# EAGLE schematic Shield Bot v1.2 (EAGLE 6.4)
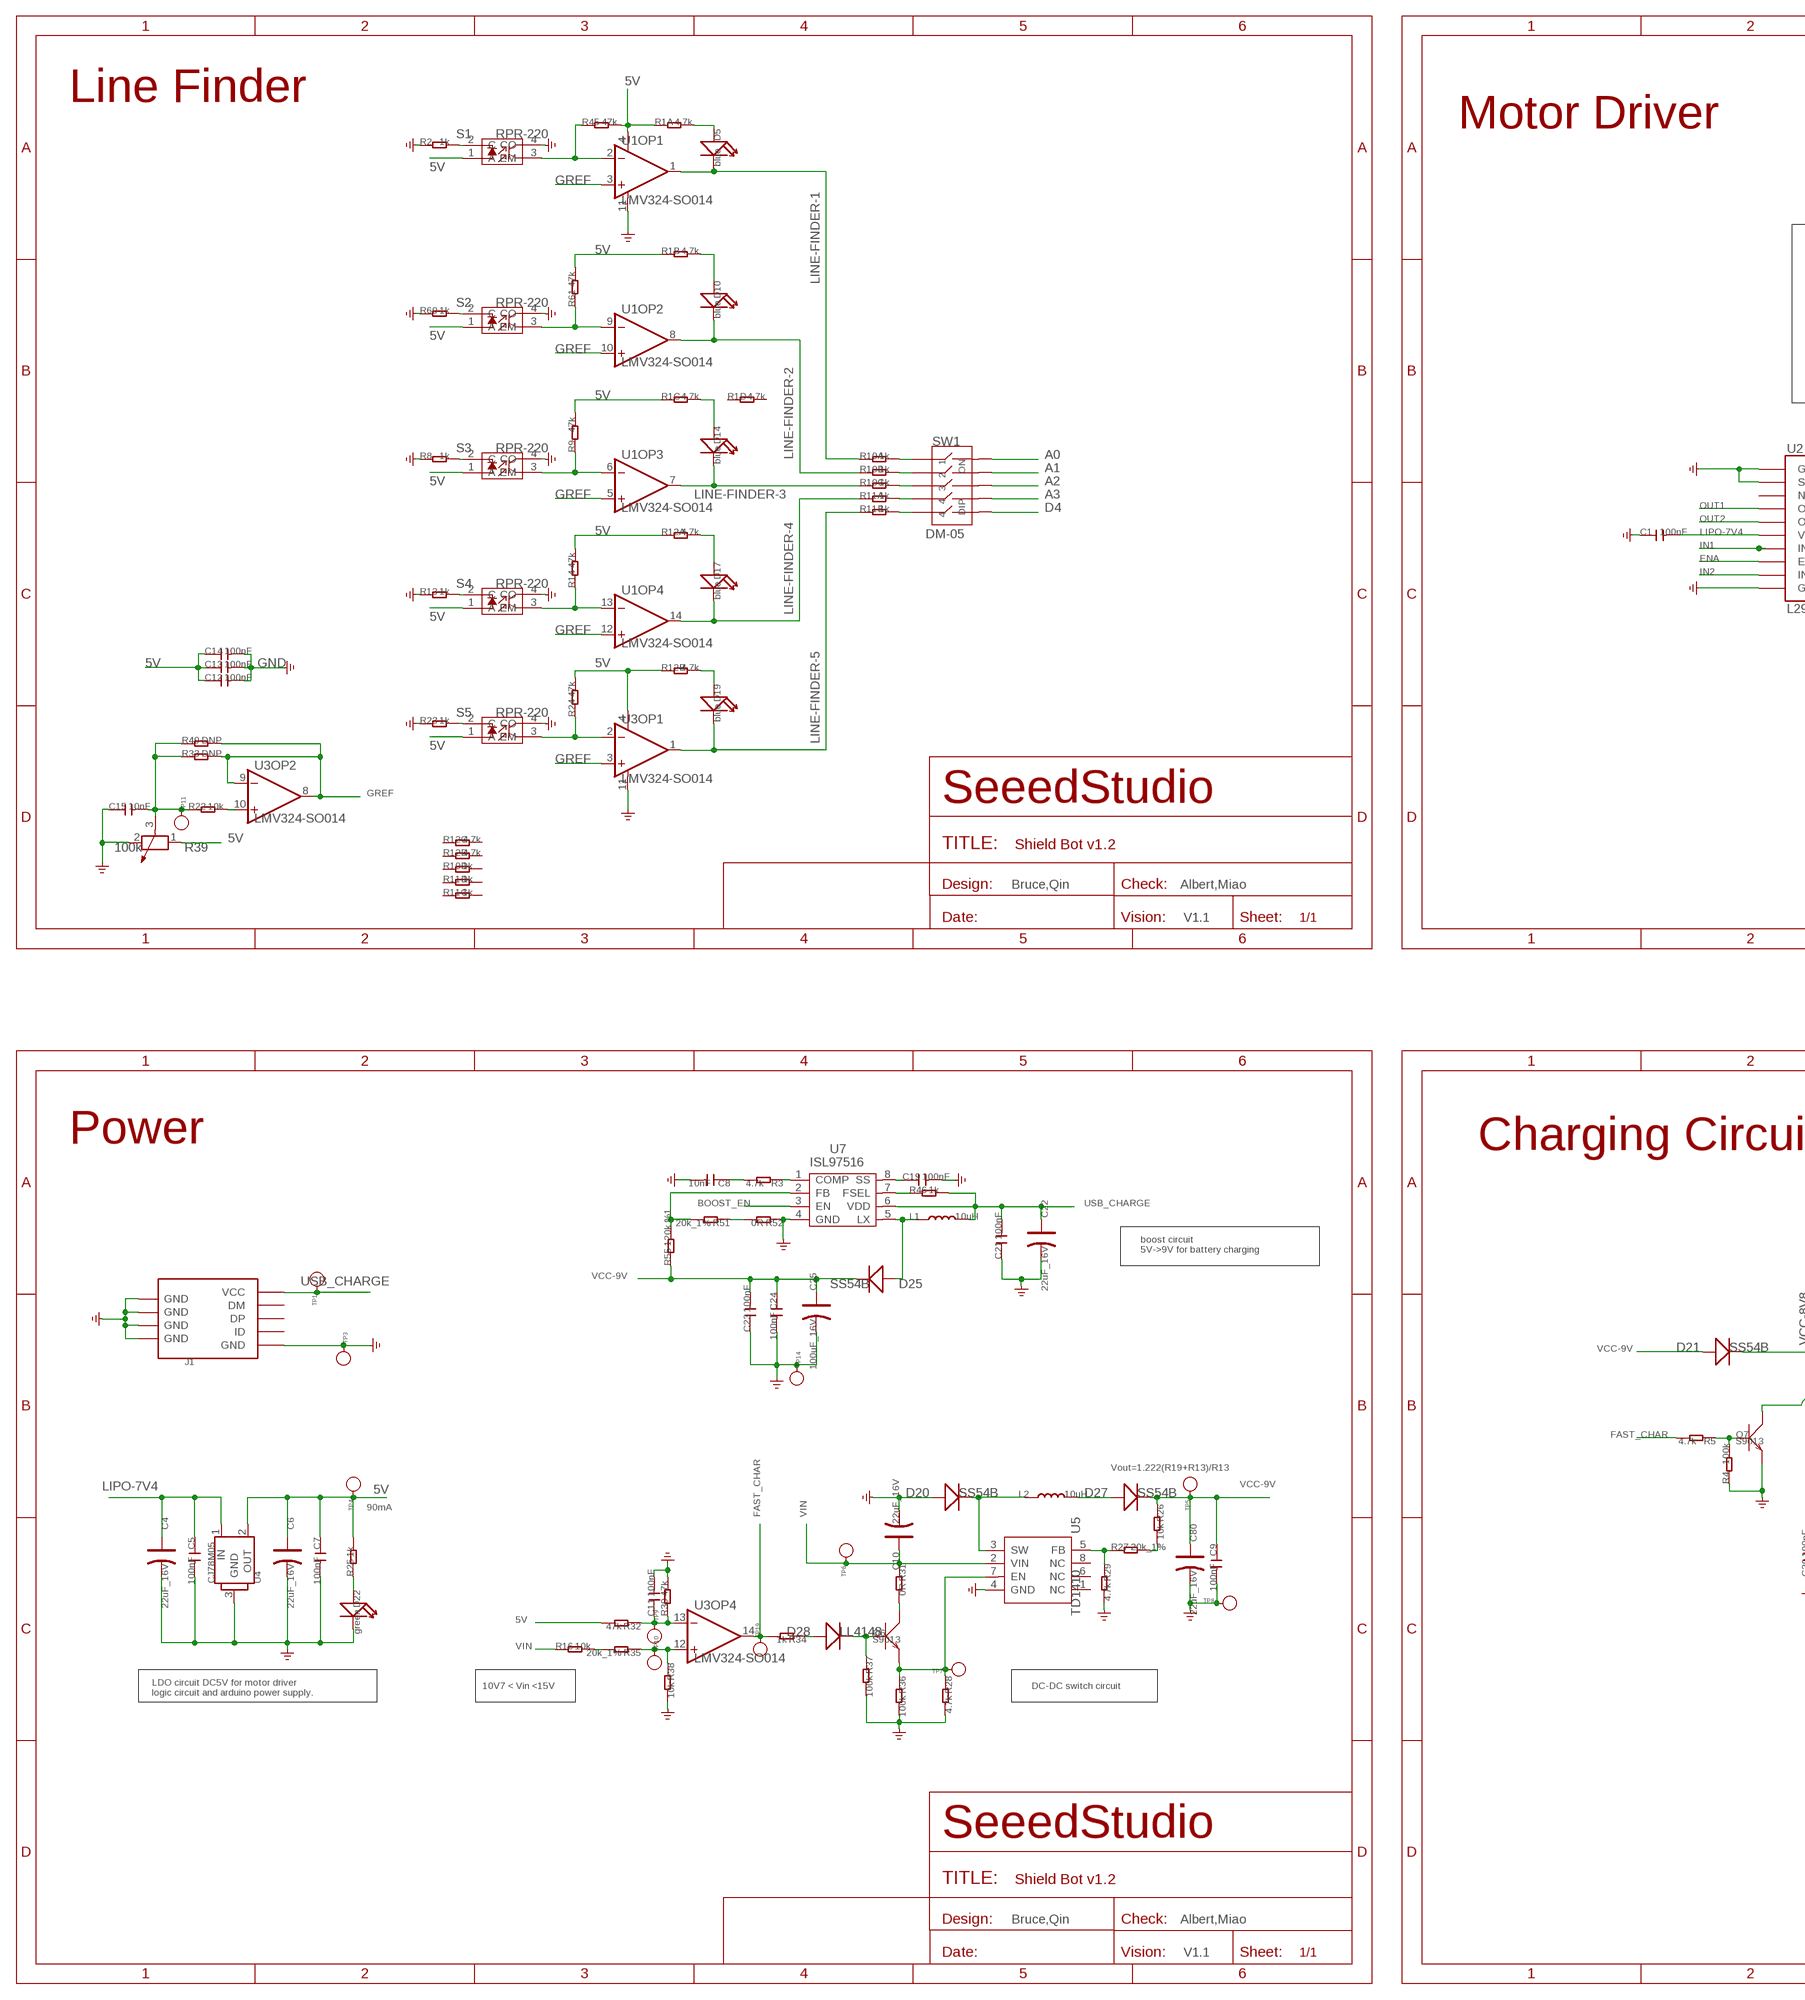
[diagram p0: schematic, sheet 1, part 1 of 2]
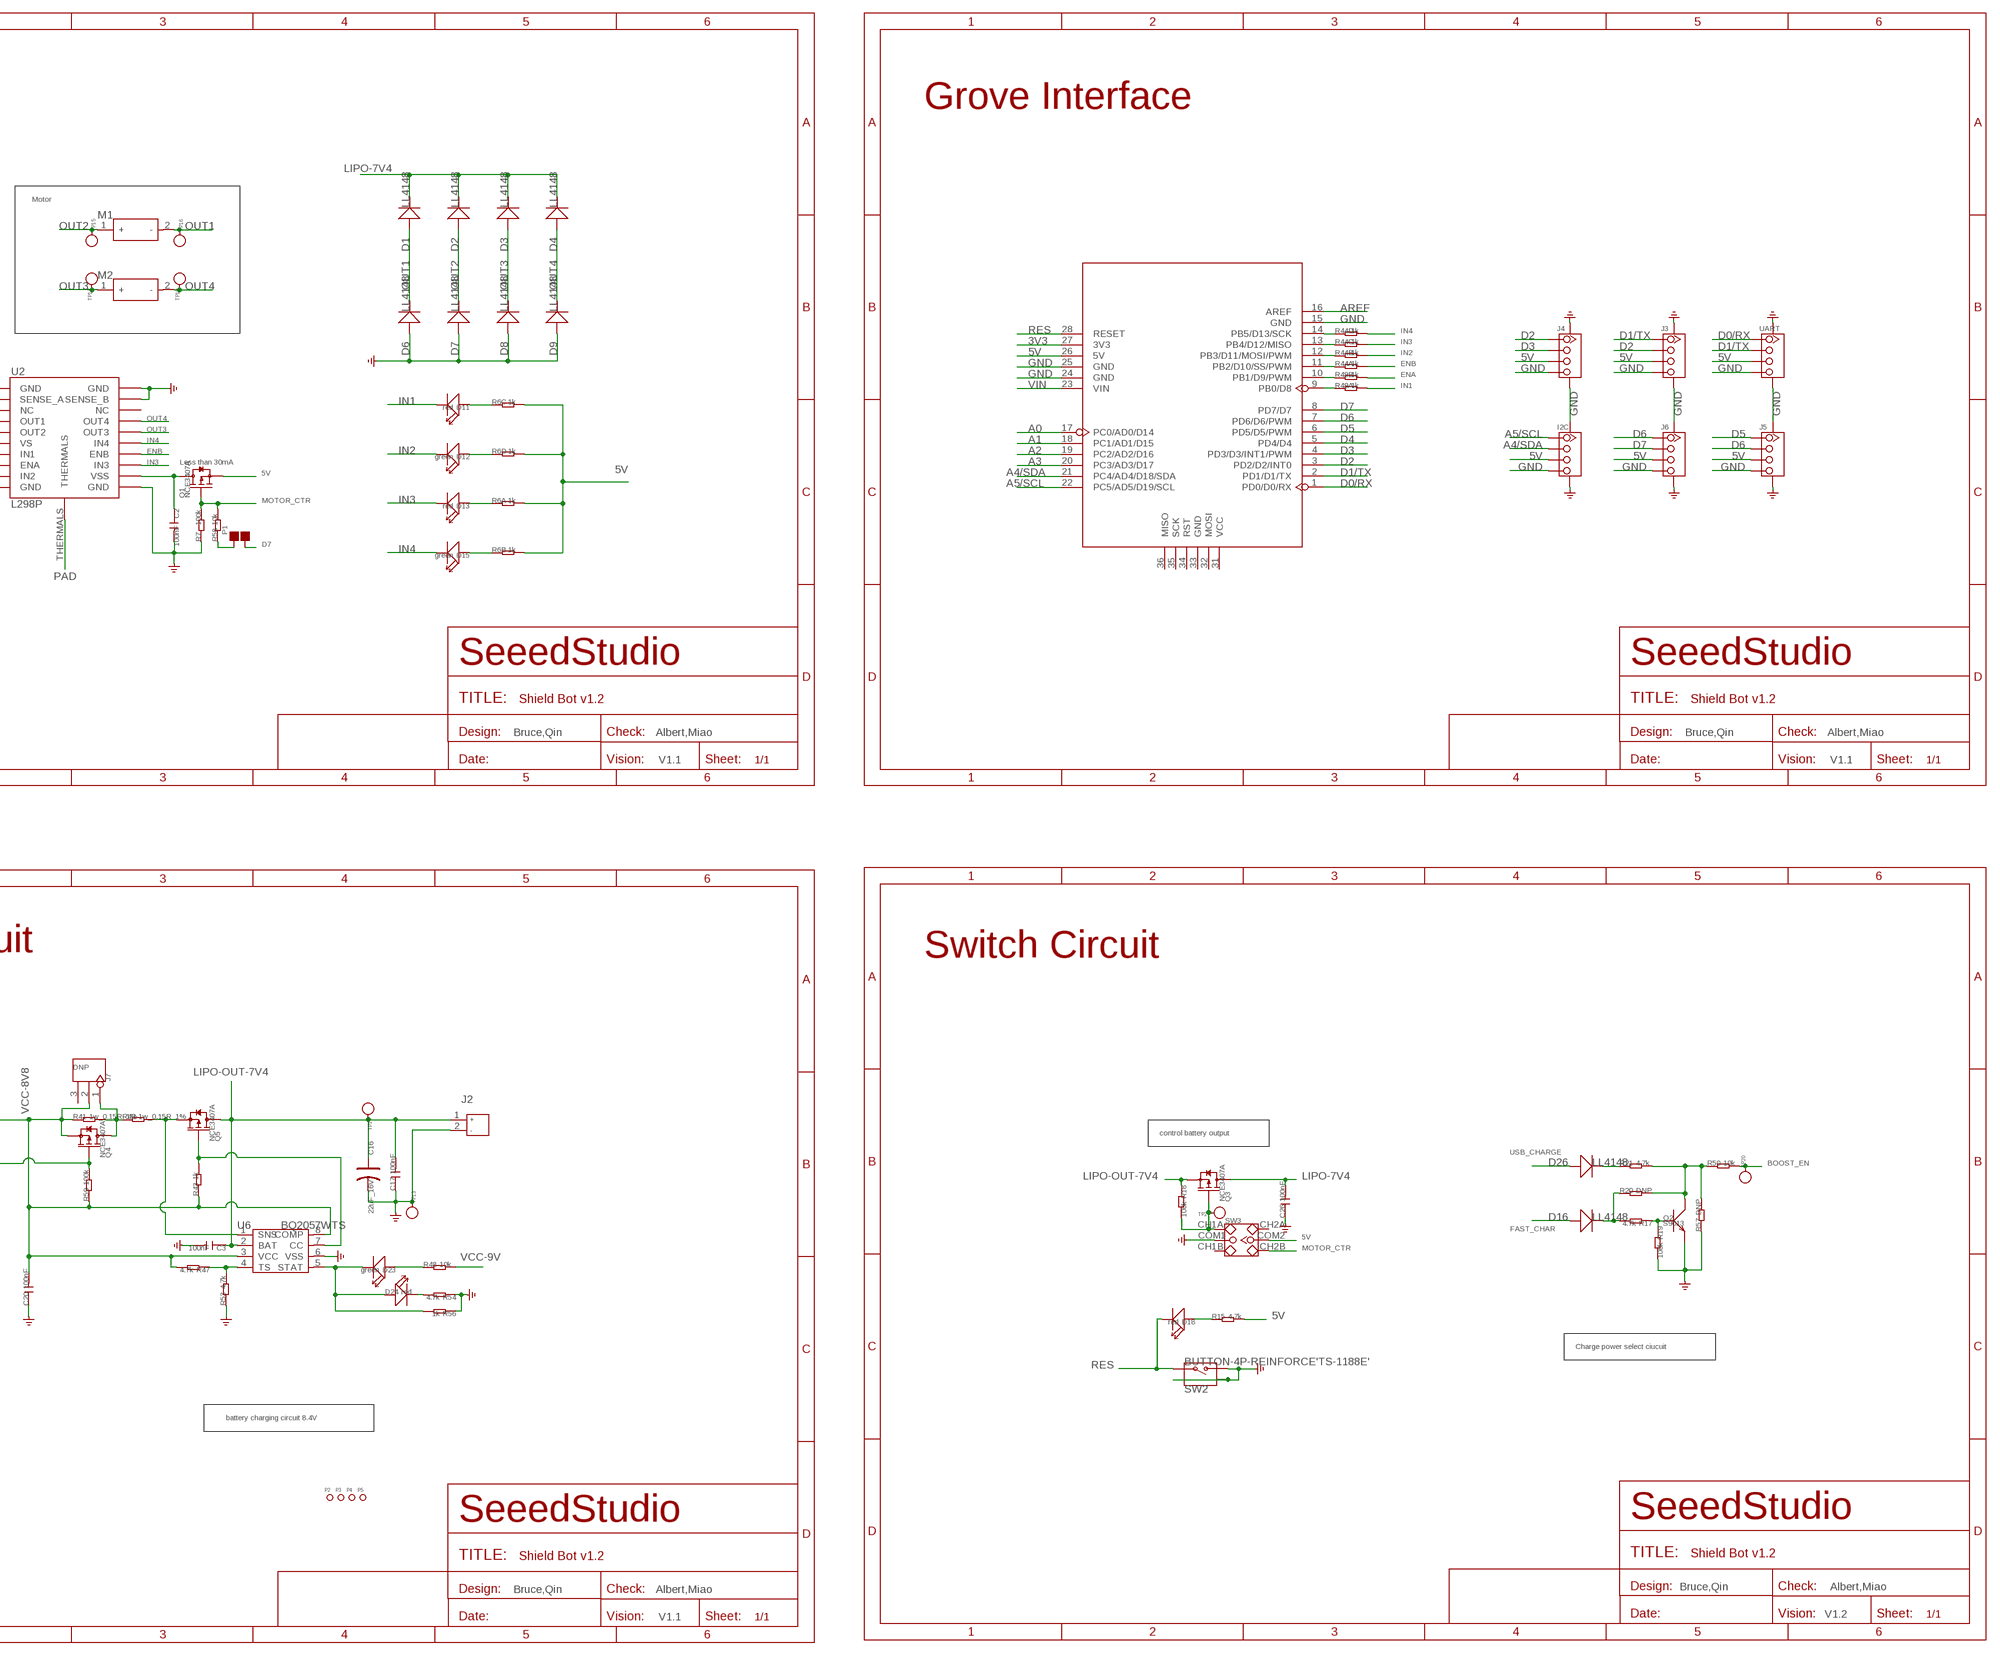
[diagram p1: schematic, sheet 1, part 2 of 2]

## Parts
C1  100nF  C-0603  [C0603]
C2  100nF  C-0603  [C0603]
C3  100nF  C-0603  [C0603]
C4  22uF_16V  CAP-AVX-B  [AVX-B]
C5  100nF  C-0603  [C0603]
C6  22uF_16V  CAP-AVX-B  [AVX-B]
C7  100nF  C-0603  [C0603]
C8  10nF  C-0603  [C0603]
C9  100nF  C-0603  [C0603]
C10  22uF_16V  CAP-AVX-B  [AVX-B]
C11  100nF  C-0603  [C0603]
C12  100nF  C-0603  [C0603]
C13  100nF  C-0603  [C0603]
C14  100nF  C-0603  [C0603]
C15  10nF  C-0603  [C0603]
C16  22uF_16V  CAP-AVX-B  [AVX-B]
C17  100nF  C-0603  [C0603]
C19  100nF  C-0603  [C0603]
C20  100nF  C-0603  [C0603]
C21  100nF  C-0603  [C0603]
C22  22uF_16V  CAP-AVX-B  [AVX-B]
C23  100nF  C-0603  [C0603]
C24  100nF  C-0603  [C0603]
C25  100uF_16V  CAP-AVX-C  [AVX-C]
C26  100nF  C-0603  [C0603]
C80  22uF_16V  CAP-AVX-B  [AVX-B]
D1  LL4148  D'1206'  [SOD123]
D2  LL4148  D'1206'  [SOD123]
D3  LL4148  D'1206'  [SOD123]
D4  LL4148  D'1206'  [SOD123]
D5  blue  LED'0603'  [LED-0603]
D6  LL4148  D'1206'  [SOD123]
D7  LL4148  D'1206'  [SOD123]
D8  LL4148  D'1206'  [SOD123]
D9  LL4148  D'1206'  [SOD123]
D10  blue  LED'0603'  [LED-0603]
D11  red  LED'0603'  [LED-0603]
D12  green  LED'0603'  [LED-0603]
D13  red  LED'0603'  [LED-0603]
D14  blue  LED'0603'  [LED-0603]
D15  green  LED'0603'  [LED-0603]
D16  LL4148  D'1206'  [SOD123]
D17  blue  LED'0603'  [LED-0603]
D18  red  LED'0603'  [LED-0603]
D19  blue  LED'0603'  [LED-0603]
D20  SS54B  D'MBRS240LT3'  [SMB]
D21  SS54B  D'MBRS240LT3'  [SMB]
D22  green  LED'0603'  [LED-0603]
D23  green  LED'0603'  [LED-0603]
D24  red  LED'0603'  [LED-0603]
D25  SS54B  D'MBRS240LT3'  [SMB]
D26  LL4148  D'1206'  [SOD123]
D27  SS54B  D'MBRS240LT3'  [SMB]
D28  LL4148  D'1206'  [SOD123]
I2C  TWIG-4P-2.0-SMD-FEMALE-REINFORCE'90D'  [4P-SMD-2.0-90D]
J1  USB-MINIUSB-5P-STRONG  [MINI-SMD-5P]
J2  JACK-JST-2P-PW'2.0'  [JST-2.0]
J3  TWIG-4P-2.0-SMD-FEMALE-REINFORCE'90D'  [4P-SMD-2.0-90D]
J4  TWIG-4P-2.0-SMD-FEMALE-REINFORCE'90D'  [4P-SMD-2.0-90D]
J5  TWIG-4P-2.0-SMD-FEMALE-REINFORCE'90D'  [4P-SMD-2.0-90D]
J6  TWIG-4P-2.0-SMD-FEMALE-REINFORCE'90D'  [4P-SMD-2.0-90D]
J7  DNP  HEADER-3P-2.54  [3P-2.54]
L1  10uH  L'0630'  [L0630]
L2  10uH  L'0630'  [L0630]
M1  MOTOR-2P-PAD  [2P-SMD-27X26]
M2  MOTOR-2P-PAD  [2P-SMD-27X26]
P1  PAD-JUMPER-2P  [2P-SMD-1.78X1.27]
P2  PAD-MARK  [ROUND-MARK-1.0]
P3  PAD-MARK  [ROUND-MARK-1.0]
P4  PAD-MARK  [ROUND-MARK-1.0]
P5  PAD-MARK  [ROUND-MARK-1.0]
Q1  NCE3407A  MOSFET-P'SI2323CDS/SI2305DS<BR>'  [SOT23]
Q2  S9013  TRANSISTOR-NPN-SOT23  [SOT23]
Q3  NCE3407A  MOSFET-P'SI2323CDS/SI2305DS<BR>'  [SOT23]
Q4  NCE3407A  MOSFET-P'SI2323CDS/SI2305DS<BR>'  [SOT23]
Q5  NCE3407A  MOSFET-P'SI2323CDS/SI2305DS<BR>'  [SOT23]
Q6  S9013  TRANSISTOR-NPN-SOT23  [SOT23]
Q7  S9013  TRANSISTOR-NPN-SOT23  [SOT23]
R1  4.7k  R-4R-1206  [1206-8-3.3X2.4]
R2  1k  R-0603  [R0603]
R3  4.7k  R-0603  [R0603]
R4  100k  R-0603  [R0603]
R5  4.7k  R-0603  [R0603]
R6  1k  R-4R-1206  [1206-8-3.3X2.4]
R7  100k  R-0603  [R0603]
R8  1k  R-0603  [R0603]
R9  47k  R-0603  [R0603]
R10  1k  R-4R-1206  [1206-8-3.3X2.4]
R11  1k  R-4R-1206  [1206-8-3.3X2.4]
R12  4.7k  R-4R-1206  [1206-8-3.3X2.4]
R13  1k  R-0603  [R0603]
R14  47k  R-0603  [R0603]
R15  4.7k  R-0603  [R0603]
R16  10k  R-0603  [R0603]
R17  4.7k  R-0603  [R0603]
R18  100k  R-0603  [R0603]
R19  100k  R-0603  [R0603]
R20  DNP  R-0603  [R0603]
R21  4.7k  R-0603  [R0603]
R22  10k  R-0603  [R0603]
R23  1k  R-0603  [R0603]
R24  47k  R-0603  [R0603]
R25  1k  R-0603  [R0603]
R26  10k  R-0603  [R0603]
R27  20k_1%  R-0603  [R0603]
R28  4.7k  R-0603  [R0603]
R29  4.7k  R-0603  [R0603]
R30  47k  R-0603  [R0603]
R31  0R  R-0603  [R0603]
R32  47k  R-0603  [R0603]
R33  DNP  R-0603  [R0603]
R34  1k  R-0603  [R0603]
R35  20k_1%  R-0603  [R0603]
R36  100k  R-0603  [R0603]
R37  100k  R-0603  [R0603]
R38  10k  R-0603  [R0603]
R39  100k  R-POTENTIOMETER'3362'  [3P-SQUA-7X6.8]
R40  DNP  R-0603  [R0603]
R41  1w_0.15R 1%  R-2512  [R2512]
R42  1w_0.15R 1%  R-2512  [R2512]
R43  1k  R-0603  [R0603]
R44  1k  R-4R-1206  [1206-8-3.3X2.4]
R45  47k  R-0603  [R0603]
R46  1k  R-0603  [R0603]
R47  4.7k  R-0603  [R0603]
R48  10k  R-0603  [R0603]
R49  1k  R-4R-1206  [1206-8-3.3X2.4]
R50  10k  R-0603  [R0603]
R51  20k_1%  R-0603  [R0603]
R52  0R  R-0603  [R0603]
R53  4.7k  R-0603  [R0603]
R54  4.7k  R-0603  [R0603]
R55  120k %1  R-0603  [R0603]
R56  1k  R-0603  [R0603]
R57  DNP  R-0603  [R0603]
R58  10k  R-0603  [R0603]
R59  100k  R-0603  [R0603]
R60  1k  R-0603  [R0603]
R61  47k  R-0603  [R0603]
S1  RPR-220  REFLECTIVE-PHOTOSENSOR-RPR-220  [4P-6.4X4.9X6.5H]
S2  RPR-220  REFLECTIVE-PHOTOSENSOR-RPR-220  [4P-6.4X4.9X6.5H]
S3  RPR-220  REFLECTIVE-PHOTOSENSOR-RPR-220  [4P-6.4X4.9X6.5H]
S4  RPR-220  REFLECTIVE-PHOTOSENSOR-RPR-220  [4P-6.4X4.9X6.5H]
S5  RPR-220  REFLECTIVE-PHOTOSENSOR-RPR-220  [4P-6.4X4.9X6.5H]
SW1  DM-05  SWITCH-KM-05-10P  [10P-SMD-14.2X6.8]
SW2  BUTTON-4P-REINFORCE'TS-1188E'  [4P-SMD-7X3.5X3.5H]
SW3  SWITCH-2CH-6P'90D'  [6P-2CH-2.54-9.0X3.6-90D]
TP1  PAD-TEST-POINT-CIRCLE'4545'  [TP_4545]
TP2  PAD-TEST-POINT-CIRCLE'4545'  [TP_4545]
TP3  PAD-TEST-POINT-CIRCLE'4545'  [TP_4545]
TP4  PAD-TEST-POINT-CIRCLE'4545'  [TP_4545]
TP5  PAD-TEST-POINT-CIRCLE'4545'  [TP_4545]
TP6  PAD-TEST-POINT-CIRCLE'4545'  [TP_4545]
TP7  PAD-TEST-POINT-CIRCLE'4545'  [TP_4545]
TP8  PAD-TEST-POINT-CIRCLE'4545'  [TP_4545]
TP9  PAD-TEST-POINT-CIRCLE'4545'  [TP_4545]
TP10  PAD-TEST-POINT-CIRCLE'4545'  [TP_4545]
TP11  PAD-TEST-POINT-CIRCLE'4545'  [TP_4545]
TP12  PAD-TEST-POINT-CIRCLE'4545'  [TP_4545]
TP13  PAD-TEST-POINT-CIRCLE'4545'  [TP_4545]
TP14  PAD-TEST-POINT-CIRCLE'4545'  [TP_4545]
TP15  PAD-TEST-POINT-CIRCLE'4545'  [TP_4545]
TP16  PAD-TEST-POINT-CIRCLE'4545'  [TP_4545]
TP17  PAD-TEST-POINT-CIRCLE'4545'  [TP_4545]
TP18  PAD-TEST-POINT-CIRCLE'4545'  [TP_4545]
TP19  PAD-TEST-POINT-CIRCLE'4545'  [TP_4545]
TP20  PAD-TEST-POINT-CIRCLE'4545'  [TP_4545]
U1  LMV324-SO014  [SO014]
U2  L298P  L298_BRIDGE_DRIVER  [POWERSO20]
U3  LMV324-SO014  [SO014]
U4  CJ78M05  78M05-TO252  [TO252]
U5  TD1410  [SOP8]
U6  BQ2057WTS  BQ2057WPW  [TSSOP8]
U7  ISL97516  [MSOP8]
U8  ARDUINO  [ARDUINO]
UART  TWIG-4P-2.0-SMD-FEMALE-REINFORCE'90D'  [4P-SMD-2.0-90D]

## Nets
3V3: U8.27(3V3)
5V: C6.+ C7.1 C12.1 C13.1 C14.1 I2C.3 J3.3 J4.3 J5.3 J6.3 Q1.2(S) R1.1 R1.2 R1.3 R6.5 R6.6 R6.7 R6.8 R9.2 R12.1 R12.2 R14.2 R15.2 R24.2 R25.2 R32.2 R39.1 R45.2 R61.2 S1.1(A) S2.1(A) S3.1(A) S4.1(A) S5.1(A) SW3.COM2 TP4.T U1.4(OP1:V+) U3.4(OP1:V+) U4.2(OUT) U8.26(5V) UART.3
A0: SW1.10 U8.17(PC0/AD0/D14)
A1: SW1.9 U8.18(PC1/AD1/D15)
A2: SW1.8 U8.19(PC2/AD2/D16)
A3: SW1.7 U8.20(PC3/AD3/D17)
A4/SDA: I2C.2 U8.21(PC4/AD4/D18/SDA)
A5/SCL: I2C.1 U8.22(PC5/AD5/D19/SCL)
AREF: U8.16(AREF)
BOOST_EN: R50.2 TP20.T U7.3(EN)
D0/RX: U8.1(PD0/D0/RX) UART.1
D1/TX: J3.1 U8.2(PD1/D1/TX) UART.2
D2: J3.2 J4.1 U8.3(PD2/D2/INT0)
D3: J4.2 U8.4(PD3/D3/INT1/PWM)
D4: SW1.6 U8.5(PD4/D4)
D5: J5.1 U8.6(PD5/D5/PWM)
D6: J5.2 J6.1 U8.7(PD6/D6/PWM)
D7: J6.2 P1.1 U8.8(PD7/D7)
ENA: R49.7 U2.P$8(ENA)
ENB: R44.8 U2.P$14(ENB)
FAST_CHAR: D16.+ R5.2 R34.2 TP19.T U3.14(OP4:OUT)
GND: C1.1 C2.2 C3.2 C4.- C5.2 C6.- C7.2 C8.2 C9.2 C10.- C11.2 C12.2 C13.2 C14.2 C15.1 C16.- C17.1 C19.2 C20.1 C21.1 C22.- C23.1 C24.2 C25.- C26.1 C80.- D6.+ D7.+ D8.+ D9.+ D20.+ D22.- I2C.4 I2C.SS1 I2C.SS2 J1.5(GND) J1.GND@1(GND) J1.GND@2(GND) J1.GND@3(GND) J1.GND@4(GND) J2.2 J3.4 J3.SS1 J3.SS2 J4.4 J4.SS1 J4.SS2 J5.4 J5.SS1 J5.SS2 J6.4 J6.SS1 J6.SS2 Q2.2(E) Q7.2(E) R2.1 R4.1 R7.1 R8.1 R13.1 R19.2 R23.1 R28.2 R29.2 R30.2 R36.2 R37.2 R38.2 R39.2 R52.1 R53.1 R54.1 R56.1 R57.1 R60.1 S1.4(CO) S2.4(CO) S3.4(CO) S4.4(CO) S5.4(CO) SW2.2 SW2.S1 SW2.S2 SW3.COM1 TP3.T TP8.T TP13.T TP14.T U1.11(OP1:V-) U2.P$1(GND) U2.P$2(SENSE_A) U2.P$10(GND) U2.P$11(GND) U2.P$19(SENSE_B) U2.P$20(GND) U3.11(OP1:V-) U4.3(GND) U5.4(GND) U6.6(VSS) U7.4(GND) U8.15(GND) U8.24(GND) U8.25(GND) UART.4 UART.SS1 UART.SS2
GREF: R33.2 R40.2 U1.3(OP1:IN+) U1.5(OP3:IN+) U1.10(OP2:IN+) U1.12(OP4:IN+) U3.3(OP1:IN+) U3.8(OP2:OUT) U3.9(OP2:IN-)
IN1: D11.- R49.8 U2.P$7(IN1)
IN2: D12.- R44.7 U2.P$9(IN2)
IN3: D13.- R44.6 U2.P$13(IN3)
IN4: D15.- R44.5 U2.P$15(IN4)
LINE-FINDER-1: D5.- R10.1 U1.1(OP1:OUT)
LINE-FINDER-2: D10.- R10.2 U1.8(OP2:OUT)
LINE-FINDER-3: D14.- R10.3 U1.7(OP3:OUT)
LINE-FINDER-4: D17.- R11.1 U1.14(OP4:OUT)
LINE-FINDER-5: D19.- R11.2 U3.1(OP1:OUT)
LIPO-7V4: C1.2 C4.+ C5.1 C26.2 D1.- D2.- D3.- D4.- Q3.3(D) U2.P$6(VS) U4.1(IN)
LIPO-OUT-7V4: C3.1 C16.+ C17.2 J2.1 Q3.2(S) Q5.3(D) R18.1 TP12.T U6.2(BAT)
MOTOR_CTR: Q1.1(G) R7.2 R58.2 SW3.CH2B
N$1: D15.+ R6.2
N$2: R45.1 S1.3(EM) U1.2(OP1:IN-)
N$3: R61.1 S2.3(EM) U1.9(OP2:IN-)
N$4: D10.+ R1.7
N$5: R2.2 S1.2(C)
N$6: R60.2 S2.2(C)
N$7: D13.+ R6.1
N$8: R9.1 S3.3(EM) U1.6(OP3:IN-)
N$9: D14.+ R1.6
N$10: R8.2 S3.2(C)
N$11: D12.+ R6.4
N$12: D5.+ R1.8
N$13: R13.2 S4.2(C)
N$14: D17.+ R12.8
N$15: R10.8 SW1.1
N$16: R26.2 R27.2
N$17: R10.7 SW1.2
N$18: D19.+ R12.7
N$19: R23.2 S5.2(C)
N$20: R24.1 S5.3(EM) U3.2(OP1:IN-)
N$21: R10.6 SW1.3
N$22: R11.8 SW1.4
N$23: R11.7 SW1.5
N$24: P1.2 R58.1
N$25: D18.+ R15.1
N$26: Q2.1(B) R17.1 R19.1
N$27: R46.1 U7.7(FSEL)
N$28: D11.+ R6.3
N$29: J7.1 Q4.3(D) R41.2 R42.1
N$30: R16.2 R35.2
N$31: D22.+ R25.1
N$32: Q5.2(S) R42.2 U6.1(SNS)
N$33: R14.1 S4.3(EM) U1.13(OP4:IN-)
N$34: D26.- R21.1
N$35: Q5.1(G) R43.2 U6.7(CC)
N$36: D24.- R54.2
N$37: R47.1 R53.2 U6.4(TS)
N$38: D23.- D24.+ R56.2 U6.5(STAT)
N$39: D23.+ R48.1
N$40: D28.- Q6.1(B) R37.1
N$41: C19.1 U7.8(SS)
N$42: R51.2 R55.2 U7.2(FB)
N$43: D25.+ L1.1 U7.5(LX)
N$44: R3.1 U7.1(COMP)
N$45: C8.1 R3.2
N$46: Q2.3(C) R20.2 R21.2 R50.1 R57.2
N$47: R35.1 R38.1 TP10.T U3.12(OP4:IN+)
N$48: D16.- R17.2 R20.1
N$49: Q3.1(G) R18.2 SW3.CH1A TP2.T
N$50: C11.1 R30.1 R32.1 TP9.T U3.13(OP4:IN-)
N$51: R51.1 R52.2
N$54: Q6.3(C) R31.2
N$55: D20.- L2.1 U5.3(SW)
N$56: C2.1 Q1.3(D) U2.P$12(VSS)
N$57: R27.1 R29.1 U5.5(FB)
N$58: R22.2 U3.10(OP2:IN+)
N$59: C15.2 R22.1 R33.1 R39.3 R40.1 TP11.T
N$61: R44.4 U8.14(PB5/D13/SCK)
N$62: R44.3 U8.13(PB4/D12/MISO)
N$63: R44.2 U8.12(PB3/D11/MOSI/PWM)
N$64: R44.1 U8.11(PB2/D10/SS/PWM)
N$65: R49.2 U8.10(PB1/D9/PWM)
N$66: R49.1 U8.9(PB0/D8)
N$70: Q6.2(E) R28.1 R36.1 TP7.T U5.7(EN)
N$71: D27.+ L2.2
N$72: Q4.1(G) Q7.3(C) R59.2
N$73: Q7.1(B) R4.2 R5.1
N$74: D28.+ R34.1
OUT1: D1.+ D6.- M1.2(-) TP16.T U2.P$4(OUT1)
OUT2: D2.+ D7.- M1.1(+) TP15.T U2.P$5(OUT2)
OUT3: D3.+ D8.- M2.1(+) TP17.T U2.P$16(OUT3)
OUT4: D4.+ D9.- M2.2(-) TP18.T U2.P$17(OUT4)
PAD: U2.THERMALS
RES: D18.- SW2.1 U8.28(RESET)
USB_CHARGE: C21.2 C22.+ D26.+ J1.1(VCC) L1.2 R46.2 TP1.T U7.6(VDD)
VCC-8V8: C20.2 D21.- J7.2 Q4.2(S) R41.1 R43.1 R47.2 R59.1 U6.3(VCC) U6.8(COMP)
VCC-9V: C9.1 C23.2 C24.1 C25.+ C80.+ D21.+ D25.- D27.- R26.1 R48.2 R55.1 TP5.T
VIN: C10.+ R16.1 R31.1 TP6.T U5.2(VIN) U8.23(VIN)
Unconnected: J1.2(DM) J1.3(DP) J1.4(ID) J7.3 R1.4 R1.5 R10.4 R10.5 R11.3 R11.4 R11.5 R11.6 R12.3 R12.4 R12.5 R12.6 R49.3 R49.4 R49.5 R49.6 SW3.CH1B SW3.CH2A U2.P$3(NC) U2.P$18(NC) U3.5(OP3:IN+) U3.6(OP3:IN-) U3.7(OP3:OUT) U5.1(NC) U5.6(NC) U5.8(NC) U8.31(VCC) U8.32(MOSI) U8.33(GND) U8.34(RST) U8.35(SCK) U8.36(MISO)

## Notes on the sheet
- Line Finder
- Motor Driver | Grove Interface
- Motor
- Less than 30mA
- Bruce,Qin | Albert,Miao | Bruce,Qin | Albert,Miao | Bruce,Qin | Albert,Miao
- V1.1 | V1.1 | V1.1
- Power | Charging Circuit | Switch Circuit
- boost circuit
  5V->9V for battery charging
- control battery output
- Vout=1.222(R19+R13)/R13
- 90mA
- Charge power select ciucuit
- 10V7 < Vin <15V | DC-DC switch circuit
- LDO circuit DC5V for motor driver 
  logic circuit and arduino power supply.
- battery charging circuit 8.4V
- Bruce,Qin | Albert,Miao | Bruce,Qin | Albert,Miao | Bruce,Qin | Albert,Miao
- V1.1 | V1.1 | V1.2

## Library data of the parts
C1-C3 C5 C7-C9 C11-C15 C17 C19-C21 C23 C24 C26 = Discrete:C*: Ceramic Capacitors
C4 C6 C10 C16 C22 C25 C80 = Discrete:CAP*: Electrolytic Capacitors,Tantalum Capacitors and Super Capacitors
D1-D4 D6-D9 D16 D20 D21 D25-D28 = Discrete:D*
D5 D10-D15 D17-D19 D22-D24 = Discrete:LED*
I2C J3-J6 UART = Connector:TWIG-4P-2.0-SMD-FEMALE-REINFORCE
J1 = Connector:USB-MINIUSB-5P
J2 = Connector:JACK-JST-2P-PW
J7 = Connector:HEADER-3P
L1 L2 = Discrete:L*
M1 M2 = template:MOTOR-2P-PAD
P1 = Discrete:PAD-JUMPER-2P; PARTNO: DNP
P2-P5 = Discrete:PAD-MARK; PARTNO: DNP
Q1 Q3-Q5 = Discrete:MOSFET-P
Q2 Q6 Q7 = Discrete:TRANSISTOR-NPN*: NPN audion
R1 R6 R10-R12 R44 R49 = Discrete:R-4R*: Resistor Array
R2-R5 R7-R9 R13-R38 R40-R43 R45-R48 R50-R61 = Discrete:R*
R39 = Discrete:R-POTENTIOMETER*: Potentiometer
S1-S5 = Discrete:REFLECTIVE-PHOTOSENSOR-RPR-220: http://wenku.baidu.com/view/18864e7d27284b73f24250aa.html
SW1 = template:SWITCH-KM-05-10P
SW2 = Discrete:BUTTON-4P-REINFORCE: TS-1188E http://www.best-dz.com/?thread-374-2.html
SW3 = Discrete:SWITCH-2CH-6P
TP1-TP20 = Discrete:PAD-TEST-POINT-CIRCLE; PARTNO: DNP
U1 U3 = IC:LMV324: General purpose LOW Voltage, Rail-to-Rail Output Amplifiers http://www.fairchildsemi.com/ds/LM/LMV358.pdf
U2 = ICs:L298_BRIDGE_DRIVER
U4 = IC:78M05: 0.5A Three Terminal Positive Voltage Regulators http://pdf1.alldatasheet.com/datasheet-pdf/view/31368/TOSHIBA/78M05/+21_79UPLRhpDDdCDytD+/datasheet.pdf
U5 = IC:TD1410: 2A 380KHz 20V PWM Buck DC/DC Converter
U6 = template:BQ2057W: Advanced Linear Charge Management IC For Single-AND TWO-CELL Lithium-Ion And Lithium-Polymer
U7 = IC:ISL97516
U8 = moudle:ARDUINO

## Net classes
0 default: width 0.203 mm, drill 0.305 mm, clearance 0.127 mm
